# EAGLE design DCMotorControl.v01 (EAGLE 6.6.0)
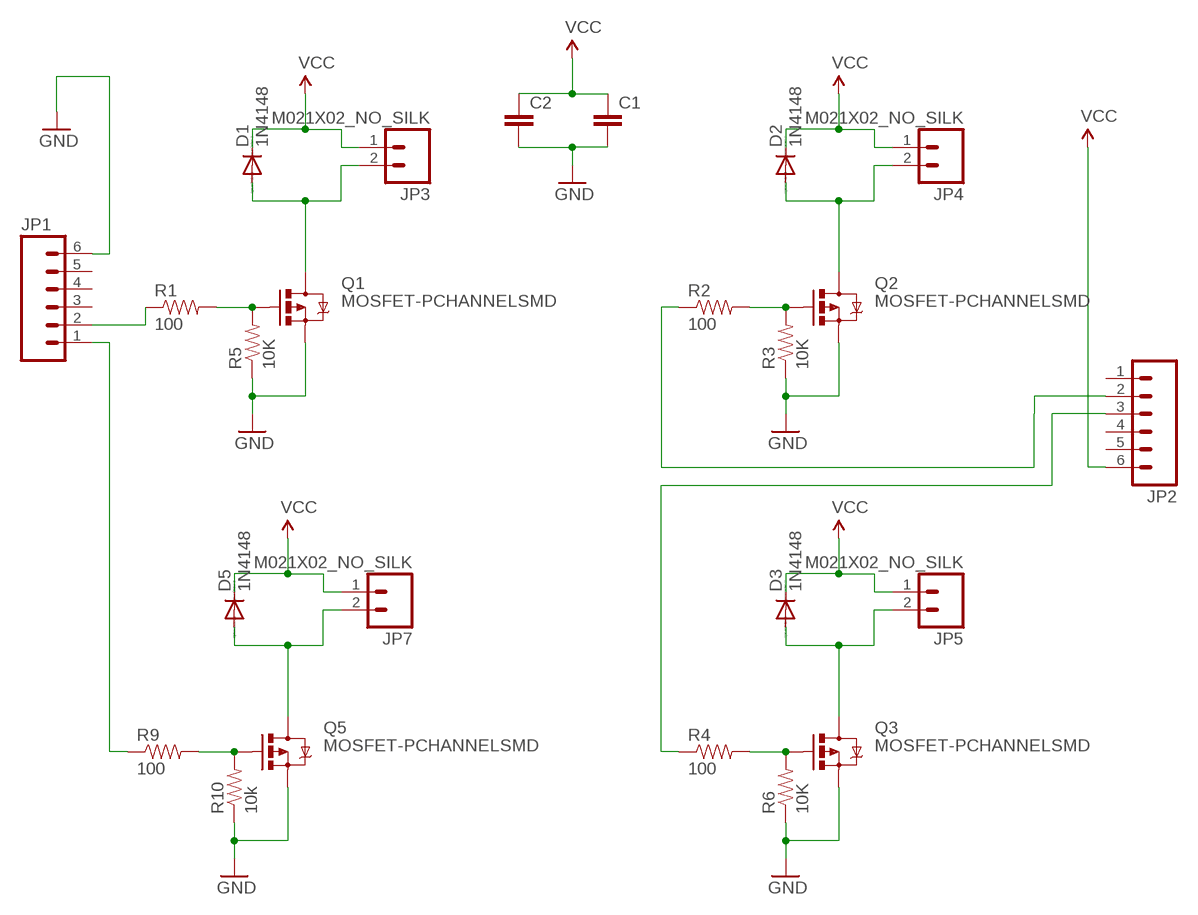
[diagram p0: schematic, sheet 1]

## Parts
C1  CAP0805  [0805]
C2  CAP0805  [0805]
D1  1N4148  DIODE-SOD323-R  [SOD323-R]
D2  1N4148  DIODE-SOD323-R  [SOD323-R]
D3  1N4148  DIODE-SOD323-R  [SOD323-R]
D5  1N4148  DIODE-SOD323-R  [SOD323-R]
JP1  M06NO_SILK  [1X06_NO_SILK]
JP2  M06NO_SILK  [1X06_NO_SILK]
JP3  M021X02_NO_SILK  [1X02_NO_SILK]
JP4  M021X02_NO_SILK  [1X02_NO_SILK]
JP5  M021X02_NO_SILK  [1X02_NO_SILK]
JP7  M021X02_NO_SILK  [1X02_NO_SILK]
Q1  MOSFET-PCHANNELSMD  [SOT23-3]
Q2  MOSFET-PCHANNELSMD  [SOT23-3]
Q3  MOSFET-PCHANNELSMD  [SOT23-3]
Q5  MOSFET-PCHANNELSMD  [SOT23-3]
R1  100  RESISTOR0805-RES  [0805]
R2  100  RESISTOR0805-RES  [0805]
R3  10K  RESISTOR0805-RES  [0805]
R4  100  RESISTOR0805-RES  [0805]
R5  10K  RESISTOR0805-RES  [0805]
R6  10K  RESISTOR0805-RES  [0805]
R9  100  RESISTOR0805-RES  [0805]
R10  10k  RESISTOR0805-RES  [0805]

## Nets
GND: C1.2 C2.2 JP1.6 Q1.2(S) Q2.2(S) Q3.2(S) Q5.2(S) R3.1 R5.1 R6.1 R10.1
N$1: D1.A JP3.2 Q1.3(D)
N$2: Q1.1(G) R1.2 R5.2
N$3: JP1.2 R1.1
N$4: D5.A JP7.2 Q5.3(D)
N$5: Q5.1(G) R9.2 R10.2
N$6: JP1.1 R9.1
N$7: D2.A JP4.2 Q2.3(D)
N$8: Q2.1(G) R2.2 R3.2
N$9: JP2.2 R2.1
N$10: D3.A JP5.2 Q3.3(D)
N$11: Q3.1(G) R4.2 R6.2
N$12: JP2.3 R4.1
VCC: C1.1 C2.1 D1.C D2.C D3.C D5.C JP2.6 JP3.1 JP4.1 JP5.1 JP7.1
Unconnected: JP1.3 JP1.4 JP1.5 JP2.1 JP2.4 JP2.5

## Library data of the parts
C1 C2 = SparkFun-Capacitors:CAP: Capacitor
D1-D3 D5 = diode:DIODE-: DIODE
JP1 JP2 = SparkFun-Connectors:M06: Header 6 Standard 6-pin 0.1" header. Use with straight break away headers (SKU : PRT-00116), right angle break away headers (PRT-00553), swiss pins (PRT-00743), machine pins (PRT-00117), and female headers (PRT-00115). Molex polarized connector foot print use with SKU : PRT-08094 with associated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
JP3-JP5 JP7 = SparkFun-Connectors:M02: Standard 2-pin 0.1" header. Use with
Q1-Q3 Q5 = SparkFun-DiscreteSemi:MOSFET-PCHANNEL: Generic PMOSFET IRLML2244 - TRANS-11153 (SOT-23 -20V -4.3A) (1.Gate 2.Source 3.Drain) FQP27P06 - COM-10349 (TO-220 -60V -27A) (1.Gate 2.Source 3.Drain)
R1-R6 R9 R10 = SparkFun-Passives:RESISTOR: Resistor

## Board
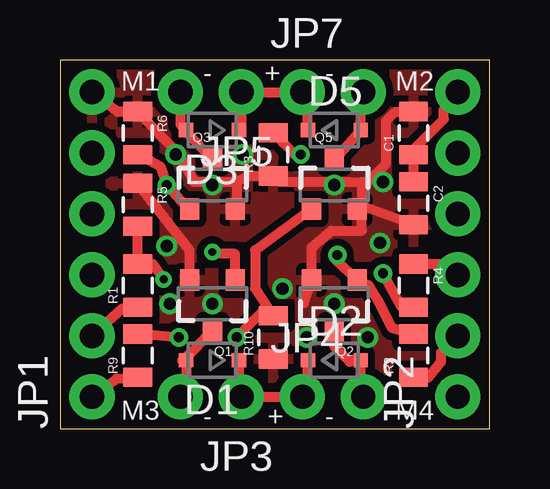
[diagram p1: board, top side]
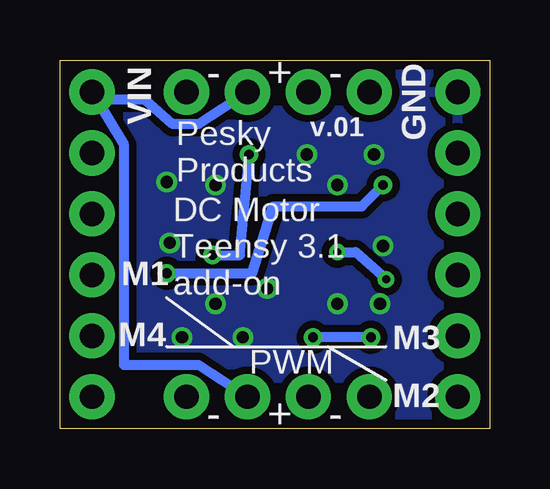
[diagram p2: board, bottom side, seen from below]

Size 17.91 x 15.37 mm. Coordinates in mm from the lower left corner, seen from the top.
Outline: 0,0 17.91,0 17.91,15.37 0,15.37 0,0
Copper layers (1*16): Top 0.0356mm / dielectric 1.5011mm / Bottom 0.0356mm
Design rules "OSHPark *": minimum track width 6mil, minimum drill 13mil, track to track 6mil, track to pad 6mil, pad to pad 6mil, via to via 6mil, smd to smd 6mil, copper to edge 15mil, drill to drill 6mil, minimum pad ring 7mil, minimum via ring 7mil, stop-mask expansion 3mil, vias tented up to drill 20mil, thermal gap 10mil

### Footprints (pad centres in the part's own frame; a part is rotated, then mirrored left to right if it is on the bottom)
0805 = smd 0.8 x 1.2: 1 -0.9,0; 2 0.9,0
SOD323-R = smd 0.6 x 0.6: A 1.1,0; C -1.1,0
1X06_NO_SILK = drill 1.016 pad 1.88: 1 0,0; 2 2.54,0; 3 5.08,0; 4 7.62,0; 5 10.16,0; 6 12.7,0
1X02_NO_SILK = drill 1.016 pad 1.88: 1 0,0; 2 2.54,0
SOT23-3 = smd 0.8 x 0.9: 1 -0.95,-1; 2 0.95,-1; 3 0,1.1

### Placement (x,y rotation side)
C1  14.73,12.32 90 top
C2  14.73,9.4 270 top
D1  6.35,2.86 180 top
D2  11.43,2.86 0 top
D3  6.35,12.45 180 top
D5  11.43,12.45 0 top
JP1  1.33,1.33 90 top
JP2  16.57,1.33 90 top
JP3  7.56,1.33 180 top
JP4  10.1,1.33 0 top
JP5  7.56,14.03 180 top
JP7  10.1,14.03 0 top
Q1  6.35,5.21 180 top
Q2  11.43,5.21 180 top
Q3  6.35,10.16 0 top
Q5  11.43,10.16 0 top
R1  3.24,5.97 90 top
R2  14.73,3.05 90 top
R3  8.89,11.43 90 top
R4  14.73,5.97 270 top
R5  3.24,9.33 270 top
R6  3.24,12.32 270 top
R9  3.24,3.05 90 top
R10  8.89,3.81 90 top

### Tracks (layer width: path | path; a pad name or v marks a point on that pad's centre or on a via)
GND  (via drill 0.51)
  Top 0.406: Q1.2 5.4,7.44 R5.1 | 1.4,13.97 2.41,13.21 R6.1 4.94,11.44 5.59,10.29 7.37,10.29 | 1.52,13.84 1.4,13.97 | 1.4,13.97 JP1.6 | 7.37,10.29 7.86,10.53 R3.1 9.14,10.28 12.05,10.28 12.57,10.29 | 7.37,10.29 7.37,9.61 Q3.2 | 12.57,10.29 12.57,9.48 Q5.2 | 10.16,5.25 Q2.2 10.48,7.56 11.3,8.26 12.57,8.26 12.57,9.35 Q5.2 | C2.2 12.66,9.26 Q5.2 | 12.57,10.29 12.83,10.29 13.59,11.05 13.59,12.83 13.97,13.21 14.59,13.21 C1.2
  other vias: 11.43,5.21 11.43,10.16 6.35,10.16 4.83,11.43 13.46,10.29 13.34,7.75 10.29,3.81 9.27,5.84 6.35,5.21 12.83,3.81 4.45,7.62 7.62,11.43 4.57,5.21
  pour Top (isolate 0.305): 0,15.37 0,0 17.91,0 17.91,15.37
  pour Bottom (isolate 0.305): 0,15.37 0,0 17.91,0 17.91,15.37
N$1
  Top 0.406: JP3.2 5.25,1.44 D1.A 5.08,2.84 5.46,3.17 5.63,3.35 Q1.3
N$2  (via drill 0.33)
  Top 0.406: Q1.1 7.3,7.29 6.43,7.29 v6.35,7.37 | R5.2 R1.2 3.88,6.86 v4.32,6.22
  Bottom 0.406: v6.35,7.37 5.59,7.37 v4.32,6.22
N$3
  Top 0.406: JP1.2 2.62,5.02 R1.1
N$4
  Top 0.406: JP7.2 12.53,13.85 D5.A 11.64,11.43 11.56,11.43 Q5.3
N$5  (via drill 0.41)
  Top 0.406: Q5.1 8.13,7.44 8.13,5.85 8.64,5.08 | 8.64,5.08 R10.2 | R9.2 3.67,3.95 3.68,3.94 v4.95,3.81 | v7.37,3.81 8.64,5.08
  Bottom 0.406: v4.95,3.81 v7.37,3.81
N$6
  Top 0.406: JP1.1 2.36,2.1 R9.1
N$7
  Top 0.406: JP4.2 12.53,1.47 D2.A 12.06,2.79 11.43,3.43 Q2.3
N$8  (via drill 0.41)
  Top 0.406: R2.2 13.84,4.19 13.25,5.33 12.87,5.97 Q2.1 11.49,7.05 v11.56,7.24 | v10.03,11.43 9.78,11.43 9.27,11.94 9.27,11.95 R3.2
  Bottom 0.406: v11.56,7.24 10.41,7.24 10.03,11.18 v10.03,11.43
N$9
  Top 0.406: R2.1 15.36,2.15 15.88,2.79 15.88,3.17 JP2.2
N$10
  Top 0.406: 6.31,11.43 6.22,11.43 Q3.3 5.25,12.36 D3.A 5.02,12.68 JP5.2
N$11  (via drill 0.41)
  Top 0.406: Q3.1 5.26,9.27 v4.45,10.16 4.19,10.92 3.74,11.18 R6.2 | R4.2 14.23,5.07 13.59,6.22 13.34,6.6 v13.46,6.48
  Bottom 0.406: v13.46,6.48 9.91,6.48 9.02,9.27 5.33,9.27 v4.45,10.16
N$12
  Top 0.406: R4.1 16.12,6.87 JP2.3
VCC
  Top 0.406: JP4.1 10.33,1.37 D2.C | D5.C 10.33,14 JP7.1 JP5.1 7.56,12.55 D3.C | JP4.1 JP3.1 7.45,1.57 D1.C | JP4.1 10.35,1.33 | C2.1 C1.1 14.8,11.7 16,12.9 16,13.33 JP2.6
  Bottom 0.406: JP7.1 12.14,12.7 13.21,12.7 14.35,13.72 16.26,13.72 JP2.6 15.24,11.81 15.24,2.67 12.14,2.67 JP4.1

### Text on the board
tPlace: - | + | - | M1 | M2 | M3 | - | + | - | M4
bPlace: GND | VIN | - | + | - | v.01 | Pesky / Products | DC Motor / Teensy 3.1 / add-on | M1 | M3 | M4 | PWM | M2 | - | + | -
